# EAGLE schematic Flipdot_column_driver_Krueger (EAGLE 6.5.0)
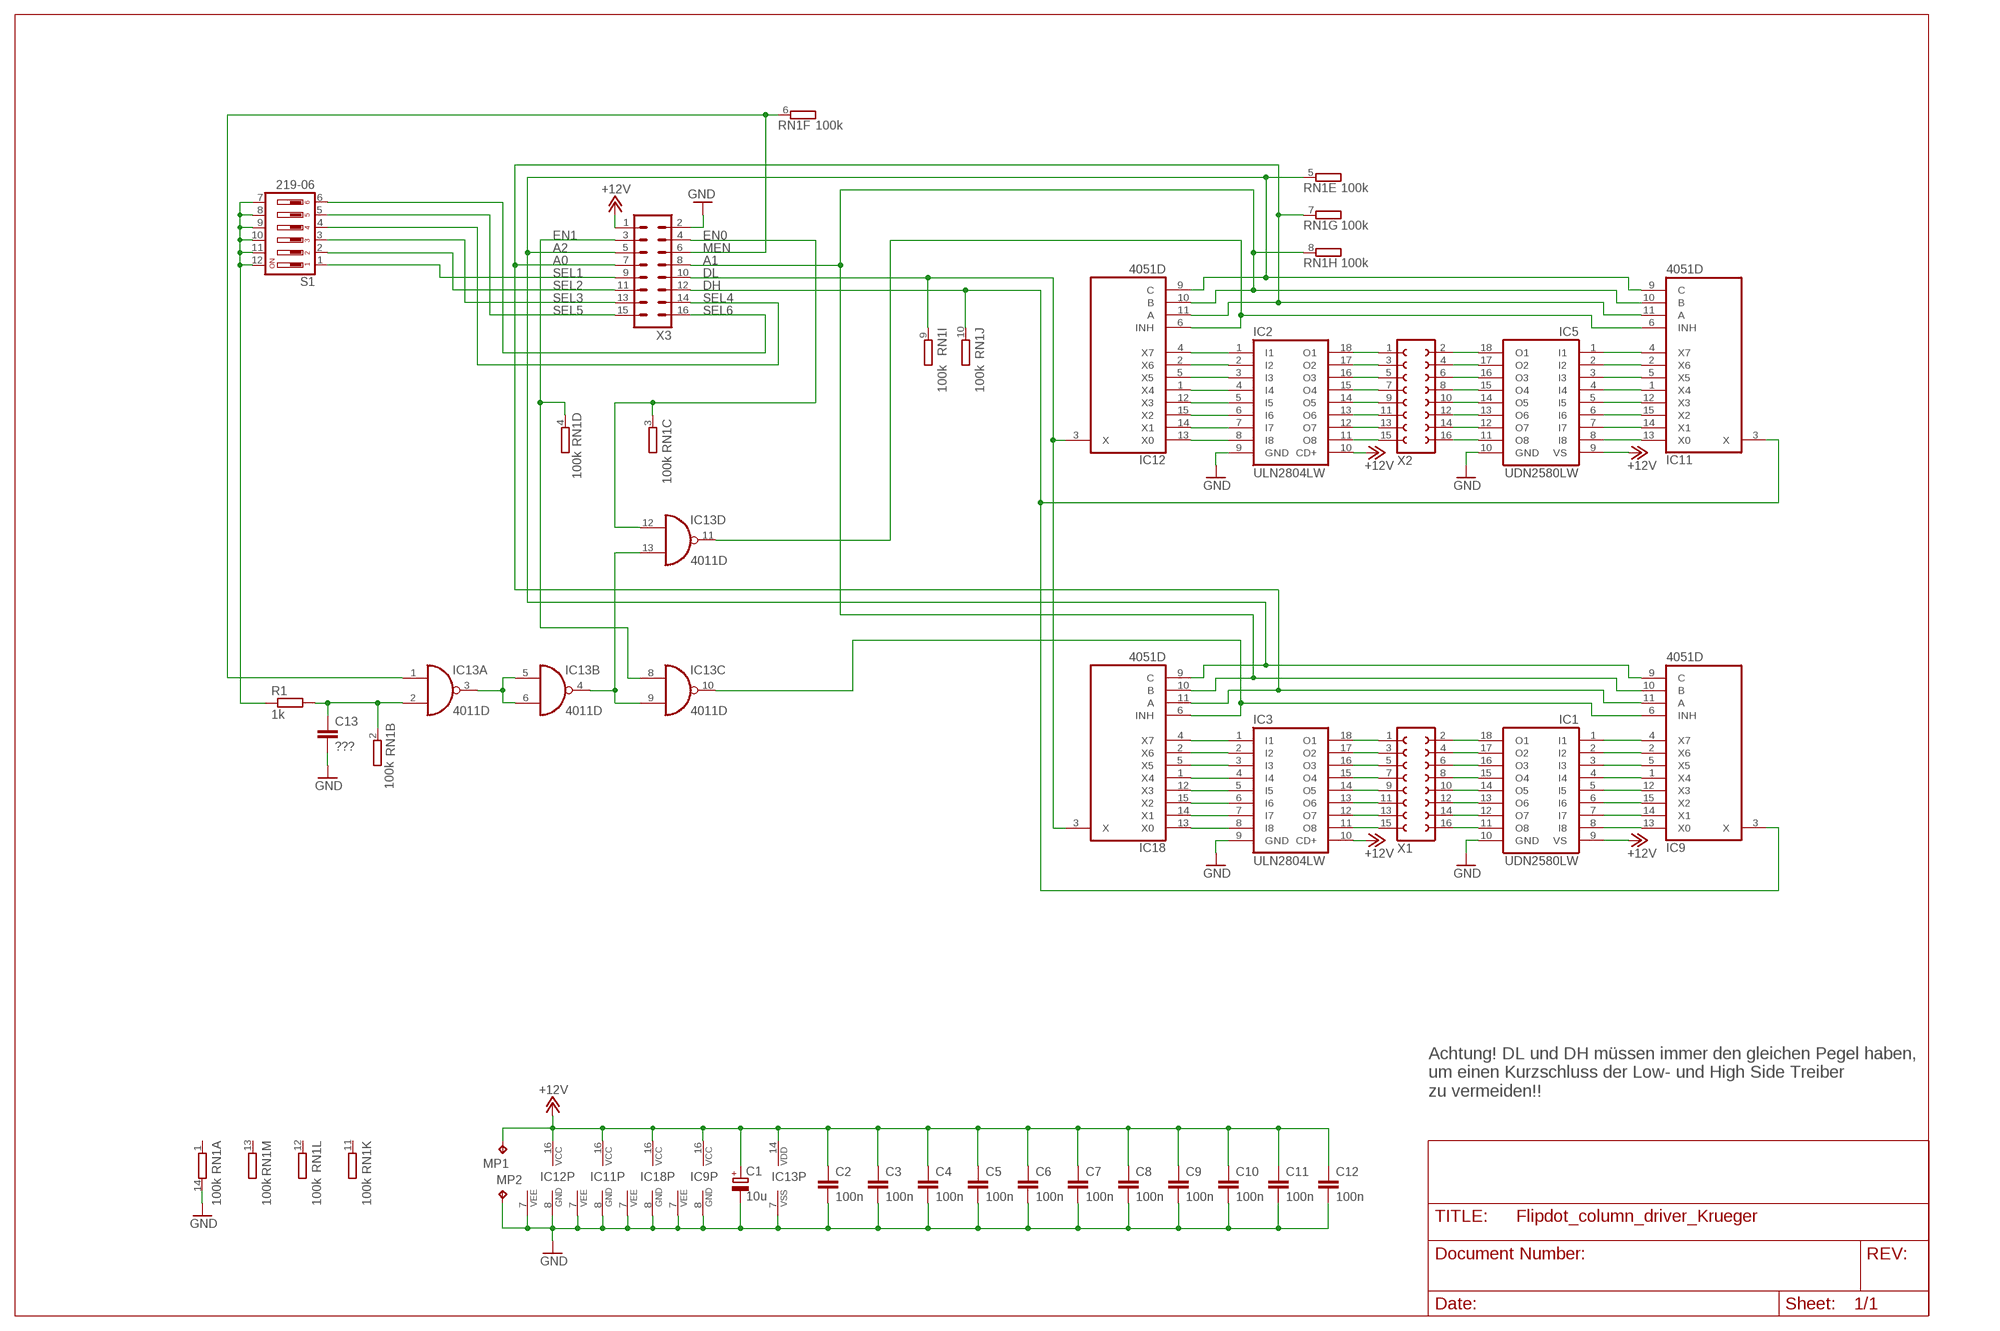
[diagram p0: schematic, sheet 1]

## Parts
C1  10u  CPOL-EUCT7343  [CT7343]
C2  100n  C-EUC1206  [C1206]
C3  100n  C-EUC1206  [C1206]
C4  100n  C-EUC1206  [C1206]
C5  100n  C-EUC1206  [C1206]
C6  100n  C-EUC1206  [C1206]
C7  100n  C-EUC1206  [C1206]
C8  100n  C-EUC1206  [C1206]
C9  100n  C-EUC1206  [C1206]
C10  100n  C-EUC1206  [C1206]
C11  100n  C-EUC1206  [C1206]
C12  100n  C-EUC1206  [C1206]
C13  ???  C-EUC1206  [C1206]
IC1  UDN2580LW  UDN2984LW  [SO18W]
IC2  ULN2804LW  ULN2803AD  [SO18W]
IC3  ULN2804LW  ULN2803AD  [SO18W]
IC5  UDN2580LW  UDN2984LW  [SO18W]
IC9  4051D  [SO16]
IC11  4051D  [SO16]
IC12  4051D  [SO16]
IC13  4011D  [SO14]
IC18  4051D  [SO16]
MP1  TPP1-08  [P1-08]
MP2  TPP1-08  [P1-08]
R1  1k  R-EU_R1206  [R1206]
RN1  100k  E13RSOMC  [SOMC14]
S1  219-06  [CTS-219-06]
X1  FE08-2  [FE08-2]
X2  FE08-2  [FE08-2]
X3  ML163ML  [3M_16L]

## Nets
+12V: C1.+ C2.1 C3.1 C4.1 C5.1 C6.1 C7.1 C8.1 C9.1 C10.1 C11.1 C12.1 IC1.9(VS) IC2.10(CD+) IC3.10(CD+) IC5.9(VS) IC9.16(VCC) IC11.16(VCC) IC12.16(VCC) IC13.14(P:VDD) IC18.16(VCC) MP1.TP X3.1
A0: IC9.11(A) IC11.11(A) IC12.11(A) IC18.11(A) RN1.7 X3.7
A1: IC9.10(B) IC11.10(B) IC12.10(B) IC18.10(B) RN1.8 X3.8
A2: IC9.9(C) IC11.9(C) IC12.9(C) IC18.9(C) RN1.5 X3.5
DH: IC9.3(X) IC11.3(X) RN1.10 X3.12
DL: IC12.3(X) IC18.3(X) RN1.9 X3.10
EN0: IC13.12(D:I0) RN1.3 X3.4
EN1: IC13.8(C:I0) RN1.4 X3.3
GND: C1.- C2.2 C3.2 C4.2 C5.2 C6.2 C7.2 C8.2 C9.2 C10.2 C11.2 C12.2 C13.2 IC1.10(GND) IC2.9(GND) IC3.9(GND) IC5.10(GND) IC9.7(VEE) IC9.8(GND) IC11.7(VEE) IC11.8(GND) IC12.7(VEE) IC12.8(GND) IC13.7(P:VSS) IC18.7(VEE) IC18.8(GND) MP2.TP RN1.14 X3.2
MEN: IC13.1(A:I0) RN1.6 X3.6
N$1: IC2.18(O1) X2.1
N$2: IC2.17(O2) X2.3
N$3: IC2.16(O3) X2.5
N$4: IC2.15(O4) X2.7
N$5: IC2.14(O5) X2.9
N$6: IC2.13(O6) X2.11
N$7: IC2.12(O7) X2.13
N$8: IC2.11(O8) X2.15
N$9: IC5.11(O8) X2.16
N$10: IC5.18(O1) X2.2
N$11: IC5.17(O2) X2.4
N$12: IC5.16(O3) X2.6
N$13: IC5.15(O4) X2.8
N$14: IC5.14(O5) X2.10
N$15: IC5.13(O6) X2.12
N$16: IC5.12(O7) X2.14
N$17: IC2.1(I1) IC12.4(X7)
N$18: IC2.2(I2) IC12.2(X6)
N$19: IC2.3(I3) IC12.5(X5)
N$20: IC2.4(I4) IC12.1(X4)
N$21: IC2.5(I5) IC12.12(X3)
N$22: IC2.6(I6) IC12.15(X2)
N$23: IC2.7(I7) IC12.14(X1)
N$24: IC2.8(I8) IC12.13(X0)
N$25: IC5.4(I4) IC11.1(X4)
N$26: IC5.2(I2) IC11.2(X6)
N$27: IC5.1(I1) IC11.4(X7)
N$28: IC5.3(I3) IC11.5(X5)
N$29: IC5.5(I5) IC11.12(X3)
N$30: IC5.8(I8) IC11.13(X0)
N$31: IC5.7(I7) IC11.14(X1)
N$32: IC5.6(I6) IC11.15(X2)
N$34: C13.1 IC13.2(A:I1) R1.2 RN1.2
N$35: IC9.6(INH) IC13.10(C:O) IC18.6(INH)
N$36: IC13.3(A:O) IC13.5(B:I0) IC13.6(B:I1)
N$39: IC13.4(B:O) IC13.9(C:I1) IC13.13(D:I1)
N$42: R1.1 S1.7 S1.8 S1.9 S1.10 S1.11 S1.12
N$45: IC3.18(O1) X1.1
N$46: IC3.17(O2) X1.3
N$47: IC3.16(O3) X1.5
N$48: IC3.15(O4) X1.7
N$49: IC3.14(O5) X1.9
N$50: IC3.13(O6) X1.11
N$51: IC3.12(O7) X1.13
N$52: IC3.11(O8) X1.15
N$53: IC1.11(O8) X1.16
N$54: IC1.18(O1) X1.2
N$55: IC1.17(O2) X1.4
N$56: IC1.16(O3) X1.6
N$57: IC1.15(O4) X1.8
N$58: IC1.14(O5) X1.10
N$59: IC1.13(O6) X1.12
N$60: IC1.12(O7) X1.14
N$61: IC3.1(I1) IC18.4(X7)
N$62: IC3.2(I2) IC18.2(X6)
N$63: IC3.3(I3) IC18.5(X5)
N$64: IC3.4(I4) IC18.1(X4)
N$65: IC3.5(I5) IC18.12(X3)
N$66: IC3.6(I6) IC18.15(X2)
N$67: IC3.7(I7) IC18.14(X1)
N$68: IC3.8(I8) IC18.13(X0)
N$69: IC1.4(I4) IC9.1(X4)
N$70: IC1.2(I2) IC9.2(X6)
N$71: IC1.1(I1) IC9.4(X7)
N$72: IC1.3(I3) IC9.5(X5)
N$73: IC1.5(I5) IC9.12(X3)
N$74: IC1.8(I8) IC9.13(X0)
N$75: IC1.7(I7) IC9.14(X1)
N$76: IC1.6(I6) IC9.15(X2)
N$77: IC11.6(INH) IC12.6(INH) IC13.11(D:O)
SEL1: S1.1 X3.9
SEL2: S1.2 X3.11
SEL3: S1.3 X3.13
SEL4: S1.4 X3.14
SEL5: S1.5 X3.15
SEL6: S1.6 X3.16
Unconnected: RN1.1 RN1.11 RN1.12 RN1.13

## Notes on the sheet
- Achtung! DL und DH müssen immer den gleichen Pegel haben,
  um einen Kurzschluss der Low- und High Side Treiber
  zu vermeiden!!

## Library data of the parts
C1 = rcl:CPOL-EU: POLARIZED CAPACITOR, European symbol
C2-C13 = rcl:C-EU: CAPACITOR, European symbol
IC1 IC5 = uln-udn:UDN298*: DRIVER ARRAY Source: Allegro Microsystems Inc. / UDN2981-UDN2984.pdf
IC2 IC3 = Brunner:ULN2803A: DRIVER ARRAY
IC9 IC11 IC12 IC18 = 40xx:4051: 8-channel ANALOG MULTIPLEXER
IC13 = 40xx:4011: Quad 2-input NAND
MP1 MP2 = testpad:TP: Test pad
R1 = rcl:R-EU_: RESISTOR, European symbol
RN1 = resistor-dil:E13R: DIL RESISTOR; MPN: SOMC140313R0GEJ; OC_FARNELL: unknown; OC_NEWARK: 48P4478
S1 = switch-dil:219-06*: Surface Mount DIP Switch Series 219 SMT CTS Electronic Components Sourc: www.ctscorp.com; OC_FARNELL: unknown; OC_NEWARK: unknown
X1 X2 = con-lsta:FE08-2: FEMALE HEADER; OC_FARNELL: unknown; OC_NEWARK: unknown
X3 = con-harting-ml:ML16: HARTING; OC_FARNELL: unknown; OC_NEWARK: unknown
